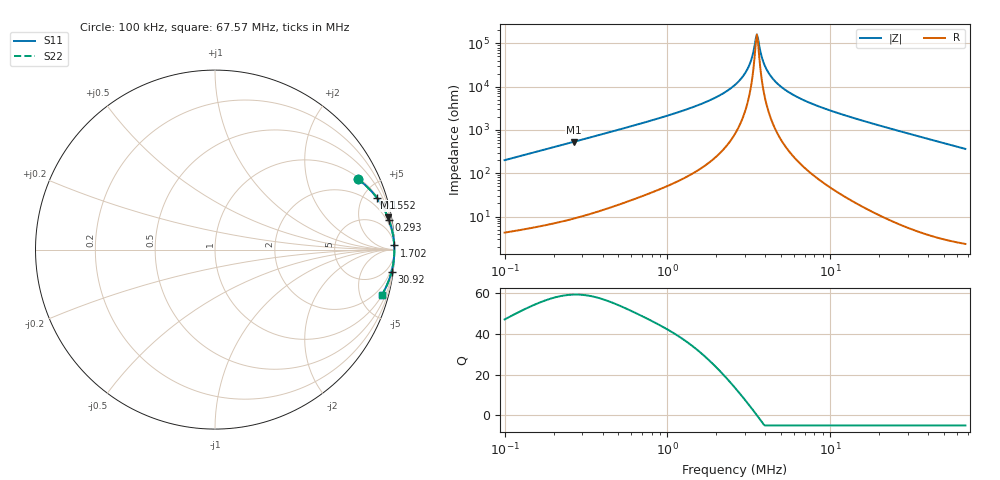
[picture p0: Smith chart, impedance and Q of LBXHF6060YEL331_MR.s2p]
! LBXHF6060YEL331_MR  S-PARAMETER MODEL  ( General Type )
! Model Generated by TAIYO YUDEN Corporation (http://www.ty-top.com)
! Version 1.0
! TAIYO YUDEN Control No. 201105NI43SB-FBB
! Copyright(c) 2020 TAIYO YUDEN CO.,LTD. All Rights Reserved.
! Product Description (link to TY-COMPAS)
! https://ds.yuden.co.jp/TYCOMPAS/or/detail?pn=LBXHF6060YEL331MMR&u=M
! Products Name : Inductors
! Characteristics :
!  Inductance : 330 uH , SRF(min) : 2.5 MHz , DC Resistance(max) : 1.872 Ohm
!  Rated Current : Saturation :550 mA , Temp Rise : 290 mA
!  Case Size : 6.0 x 6.0 / 0.236 x 0.236 [mm/inch] , Thickness : 4.5 / 0.177 [mm/inch]
!  (Conditions: Temperature = 25 degC , DC Bias Current/Voltage = 0A / 0V)
! External Node Assignments :
!  1  o---GGG---o  2
! GND o---------o GND
! Frequency Range : 0.1MHz  -  67.570357MHz  [ 402 STEP ]
# MHz S RI R 50
! Freq[MHz].  S11 Real  S11 Imag  S21 Real  S21 Imag  S12 Real  S12 Imag  S22 Real  S22 Imag
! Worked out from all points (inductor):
!   401 points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, 100 kHz to 67.57 MHz, reference 50 ohm
!   read as one part in series: L = 318 uH near 103.3 kHz
!   highest Q = 59.3 at 265.7 kHz (marker M1), where L = 318 uH
!   self-resonance near 3.542 MHz
!   S11 on the Smith chart (normalised r, x): 100 kHz: 1.09, +4.00; 155.2 kHz: 1.11, +6.20; 293 kHz: 1, +12; 1.702 MHz: 4, +87; 30.92 MHz: 1, -16; 67.57 MHz: 1.05, -7.29
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0.1  0.7954 0.3929  0.2046 -0.3929  0.2046 -0.3929  0.7954 0.3929
0.155242  0.9016 0.2888  0.0984 -0.2888  0.0984 -0.2888  0.9016 0.2888
0.265744  0.963 0.1806  0.037 -0.1806  0.037 -0.1806  0.963 0.1806
0.293028  0.9691 0.1648  0.0309 -0.1648  0.0309 -0.1648  0.9691 0.1648
0.297841  0.97 0.1623  0.03 -0.1623  0.03 -0.1623  0.97 0.1623
0.887091  0.9959 0.0533  0.00406 -0.0533  0.00406 -0.0533  0.9959 0.0533
1.701939  0.9987 0.023  0.00133 -0.023  0.00133 -0.023  0.9987 0.023
2.59943  0.9992 0.00906  0.000753 -0.00906  0.000753 -0.00906  0.9992 0.00906
2.866319  0.9993 0.00616  0.000691 -0.00616  0.000691 -0.00616  0.9993 0.00616
3.109542  0.9993 0.00378  0.000654 -0.00378  0.000654 -0.00378  0.9993 0.00378
3.265274  0.9994 0.00236  0.000638 -0.00236  0.000638 -0.00236  0.9994 0.00236
3.485115  0.9994 0.000486  0.000625 -0.000486  0.000625 -0.000486  0.9994 0.000486
3.54235  0.9994 1.69e-05  0.000622 -1.69e-05  0.000622 -1.69e-05  0.9994 1.69e-05
3.659656  0.9994 -0.000921  0.00062 0.000921  0.00062 0.000921  0.9994 -0.000921
3.842939  0.9994 -0.00233  0.000619 0.00233  0.000619 0.00233  0.9994 -0.00233
3.970199  0.9994 -0.00327  0.000622 0.00327  0.000622 0.00327  0.9994 -0.00327
4.5228  0.9993 -0.00709  0.000651 0.00709  0.000651 0.00709  0.9993 -0.00709
5.589519  0.9992 -0.0136  0.000775 0.0136  0.000775 0.0136  0.9992 -0.0136
7.742162  0.9988 -0.0249  0.0012 0.0249  0.0012 0.0249  0.9988 -0.0249
23.05932  0.991 -0.0907  0.00901 0.0907  0.00901 0.0907  0.991 -0.0907
30.91615  0.984 -0.1221  0.016 0.1221  0.016 0.1221  0.984 -0.1221
67.57036  0.9287 -0.2542  0.0713 0.2542  0.0713 0.2542  0.9287 -0.2542
